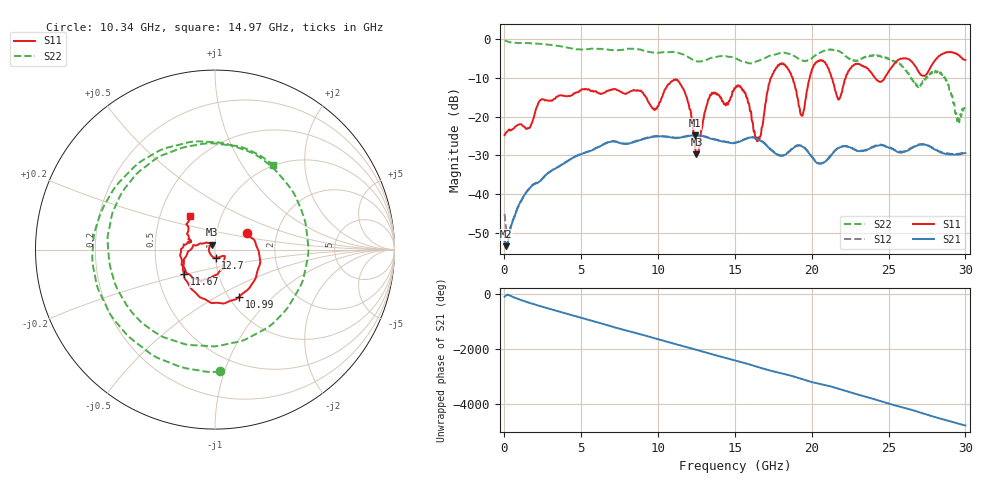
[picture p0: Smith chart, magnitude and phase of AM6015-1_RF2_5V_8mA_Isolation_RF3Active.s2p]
!Agilent Technologies,E8364B,MY43040894,A.07.50.67
!Agilent E8364B: A.07.50.67
!Date: Monday, August 13, 2018 07:03:35
!Correction: S11(Full 2 Port(1,2))
!S21(Full 2 Port(1,2))
!S12(Full 2 Port(1,2))
!S22(Full 2 Port(1,2))
!S2P File: Measurements: S11, S21, S12, S22:
# Hz S  dB  R 50
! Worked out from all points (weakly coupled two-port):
!   1601 points, 10 MHz to 30 GHz, reference 50 ohm
!   highest |S21| = -24.81 dB at 12.4 GHz (marker M1); lowest = -53.4 dB at 103.7 MHz (marker M2)
!   lowest |S11| = -29.7 dB at 12.49 GHz (marker M3), VSWR 1.07, Z = 48.1 + j2.62 ohm
!   |S11| at or under -10 dB: start of sweep to 17.33 GHz; 18.76 GHz to 19.87 GHz (1.109 GHz wide, 5.74 % of centre); 21.31 GHz to 22.21 GHz (900.1 MHz wide, 4.14 % of centre)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
!   |S22| runs from -21.5 to -0.3 dB; largest |S21 - S12| = 0.0078
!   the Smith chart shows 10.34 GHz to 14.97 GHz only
!   S11 on the Smith chart (normalised r, x): 10.34 GHz: 1.40, +0.26; 10.99 GHz: 1.12, -0.64; 11.67 GHz: 0.68, -0.20; 12.7 GHz: 1.00, -0.09; 14.97 GHz: 0.71, +0.28
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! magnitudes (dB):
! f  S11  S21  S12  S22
! 10 MHz  -24.8  -52.2  -45.1  -0.3
! 103.7 MHz  -24.1  -53.4  -48.6  -0.4
! 1.603 GHz  -23.0  -38.7  -38.6  -1.0
! 5.015 GHz  -13.0  -29.6  -29.6  -2.6
! 10.02 GHz  -17.2  -25.1  -25.0  -3.5
! 10.34 GHz  -14.0  -25.1  -25.0  -3.4
! 10.99 GHz  -10.6  -25.5  -25.3  -3.3
! 11.67 GHz  -13.1  -25.2  -25.2  -4.0
! 12.4 GHz  -27.6  -24.8  -24.7  -5.6
! 12.49 GHz  -29.7  -24.8  -24.7  -5.7
! 12.7 GHz  -26.9  -24.9  -24.8  -5.8
! 13.39 GHz  -14.3  -25.6  -25.5  -4.9
! 14.97 GHz  -12.6  -26.8  -26.7  -4.8
! 15.01 GHz  -12.7  -26.8  -26.7  -4.9
! 16.49 GHz  -26.0  -25.8  -25.7  -5.6
! 17.69 GHz  -7.4  -29.6  -29.5  -3.9
! 19.35 GHz  -19.7  -27.6  -27.5  -5.5
! 20.01 GHz  -7.9  -30.3  -30.2  -4.9
! 21.75 GHz  -15.6  -28.1  -28.0  -3.0
! 22.76 GHz  -6.6  -28.5  -28.4  -5.6
! 25.01 GHz  -8.2  -28.0  -27.8  -5.1
! 30 GHz  -5.3  -29.4  -29.2  -17.7
